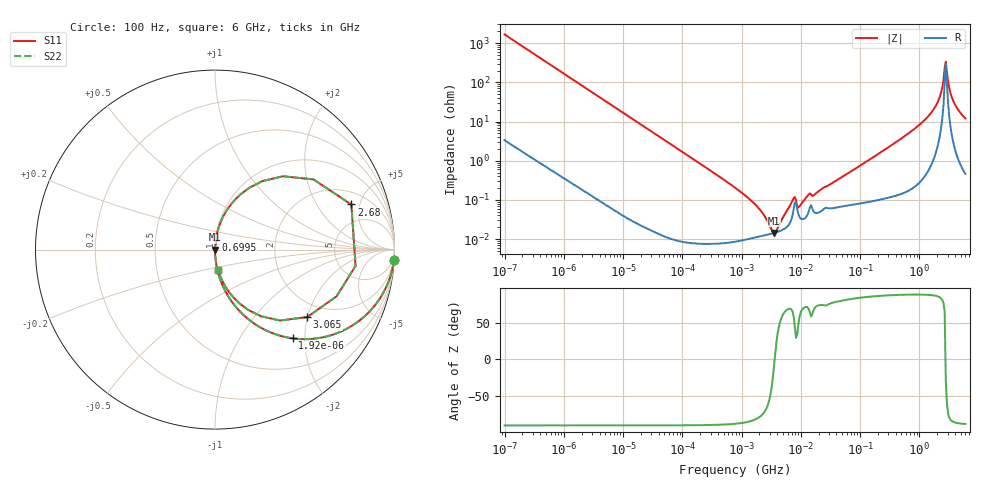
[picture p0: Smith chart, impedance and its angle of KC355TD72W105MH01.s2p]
!Murata Part Number: KC355TD72W105MH01
!These Parameters are Measured in Series Mode Connection
!Data Generated on Jun 19, 2026
!  o--ll--o
!Port1  Port2
!  o------o
!Operation Temp=25[degC], DC Bias Voltage=0[V]
!Freq. Start=100[Hz] Stop=6[GHz] 401[Steps]
# Hz S RI R 50
!Freq.(Hz) S11(Real) S11(Imag) S21(Real) S21(Imag) S12(Real) S12(Imag) S22(Real) S22(Imag)
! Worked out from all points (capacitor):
!   401 points, 100 Hz to 6 GHz, reference 50 ohm
!   read as one part in series: C = 954 nF near 109 Hz
!   lowest |Z| = 14.4 mohm at 3.55 MHz (marker M1)
!   series resonance near 3.618 MHz, so ESL is about 2 nH
!   S11 on the Smith chart (normalised r, x): 100 Hz: 1, -33; 1.92 kHz: 1.00, -1.74; 699.5 MHz: 1.00, +0.11; 2.68 GHz: 2.98, +4.16; 3.065 GHz: 1.58, -1.99; 6 GHz: 1.01, -0.24
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100  0.9963 -0.0597  0.0037 0.0597  0.0037 0.0597  0.9963 -0.0597
600  0.8855 -0.3174  0.1145 0.3174  0.1145 0.3174  0.8855 -0.3174
1920  0.432 -0.4943  0.568 0.4943  0.568 0.4943  0.432 -0.4943
2008  0.4102 -0.4908  0.5898 0.4908  0.5898 0.4908  0.4102 -0.4908
5882  0.0757 -0.2633  0.9243 0.2633  0.9243 0.2633  0.0757 -0.2633
40335  0.00187 -0.0416  0.9981 0.0416  0.9981 0.0416  0.00187 -0.0416
774597  8.97e-05 -0.00205  0.9999 0.00205  0.9999 0.00205  8.97e-05 -0.00205
1896632  0.000114 -0.000629  0.9999 0.000629  0.9999 0.000629  0.000114 -0.000629
3549919  0.000143 -1.72e-05  0.9999 1.72e-05  0.9999 1.72e-05  0.000143 -1.72e-05
7266822  0.000414 0.000872  0.9996 -0.000872  0.9996 -0.000872  0.000414 0.000872
9506416  0.000365 0.000577  0.9996 -0.000577  0.9996 -0.000577  0.000365 0.000577
1.555665e7  0.000621 0.00111  0.9994 -0.00111  0.9994 -0.00111  0.000621 0.00111
3.124326e8  0.00167 0.0228  0.9983 -0.0228  0.9983 -0.0228  0.00167 0.0228
6.994765e8  0.00465 0.0532  0.9954 -0.0532  0.9954 -0.0532  0.00465 0.0532
1.95892e9  0.0848 0.2468  0.9152 -0.2468  0.9152 -0.2468  0.0848 0.2468
2.240541e9  0.1904 0.344  0.8096 -0.344  0.8096 -0.344  0.1904 0.344
2.450438e9  0.3791 0.4087  0.6209 -0.4087  0.6209 -0.4087  0.3791 0.4087
2.679998e9  0.7597 0.2513  0.2403 -0.2513  0.2403 -0.2513  0.7597 0.2513
3.065283e9  0.5137 -0.3758  0.4863 0.3758  0.4863 0.3758  0.5137 -0.3758
3.352442e9  0.256 -0.3715  0.744 0.3715  0.744 0.3715  0.256 -0.3715
3.8344e9  0.1061 -0.2701  0.8939 0.2701  0.8939 0.2701  0.1061 -0.2701
6e9  0.0184 -0.1163  0.9816 0.1163  0.9816 0.1163  0.0184 -0.1163
